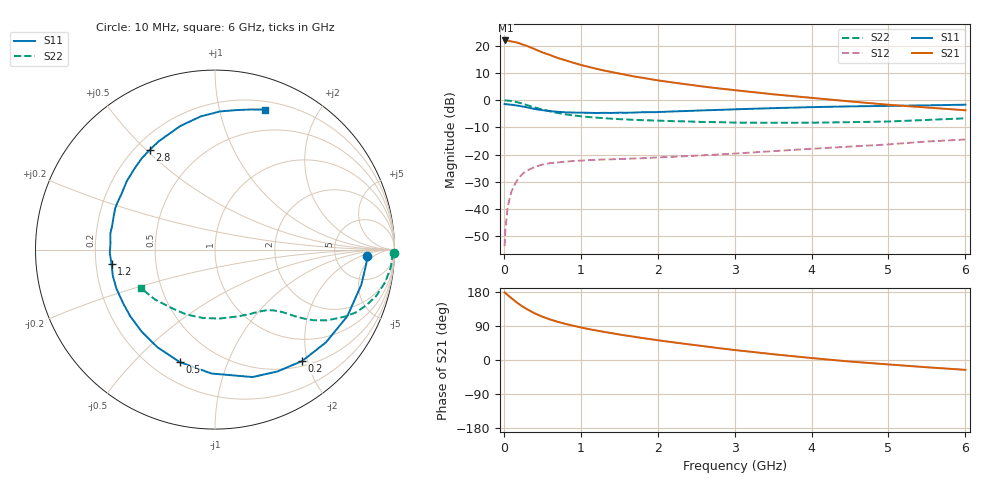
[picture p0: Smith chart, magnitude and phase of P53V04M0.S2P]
! SIEMENS Small Signal Semiconductors
! BFP183
! Si NPN RF Bipolar Junction Transistor in SOT143
! VCE = 3 V  IC = 4 mA
! Common Emitter S-Parameters:  March  1996
# GHz  S  MA  R  50
!  f  S11  S21  S12  S22
! GHz  MAG  ANG  MAG  ANG  MAG  ANG  MAG  ANG
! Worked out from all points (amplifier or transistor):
!   36 points, 10 MHz to 6 GHz, reference 50 ohm
!   highest |S21| = 21.9 dB at 20 MHz (marker M1)
!   |S21| within 3 dB of that: start of sweep to 385.1 MHz
!   unconditionally stable (mu >= 1): 1.679 GHz to 5.723 GHz
!   at 250 MHz: K = 0.18, MSG = 23.6 dB, |S12| = -26.9 dB
!   at 1.4 GHz: K = 0.87, MSG = 16.0 dB, |S12| = -21.7 dB
!   at 6 GHz: K = 0.95, MSG = 5.4 dB, |S12| = -14.4 dB
!   S11 on the Smith chart (normalised r, x): 10 MHz: 12, -3; 200 MHz: 0.58, -1.91; 500 MHz: 0.31, -0.69; 1.2 GHz: 0.27, -0.07; 2.8 GHz: 0.26, +0.51; 6 GHz: 0.28, +1.38
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0.01  0.85 -2.5  12.38 178.5  0.0021 83.7  0.9956 -1.1
0.02  0.8459 -5.6  12.48 177.0  0.0042 86.3  0.989 -2.2
0.05  0.8384 -13.5  12.36 171.2  0.0111 84.3  0.9849 -5.5
0.15  0.8058 -39.9  11.64 154.6  0.0301 69.2  0.935 -16.0
0.2  0.788 -52.0  11.08 147.1  0.0383 63.8  0.8976 -20.3
0.25  0.7629 -62.9  10.42 140.2  0.0454 58.3  0.8585 -24.1
0.3  0.7402 -73.6  9.909 134.3  0.0511 53.7  0.8139 -27.3
0.4  0.6907 -91.6  8.659 123.2  0.0594 46.0  0.7378 -32.3
0.5  0.6568 -107.3  7.544 114.4  0.066 40.4  0.676 -35.6
0.6  0.6316 -120.5  6.746 107.1  0.0701 36.2  0.6247 -37.9
0.7  0.613 -131.8  5.964 100.8  0.0722 33.4  0.582 -39.7
0.8  0.6005 -141.9  5.404 95.3  0.0745 30.7  0.5513 -41.0
1.1  0.5878 -165.5  4.1 81.7  0.0796 26.8  0.4916 -44.2
1.2  0.5818 -171.9  3.782 78.0  0.0805 26.0  0.4794 -45.3
1.5  0.5899 171.5  3.083 67.3  0.0834 25.6  0.4489 -48.6
1.7  0.5939 162.1  2.719 61.2  0.0853 25.6  0.436 -51.4
2.2  0.6223 142.1  2.109 46.7  0.0915 26.6  0.4124 -58.9
2.8  0.6648 123.0  1.642 31.1  0.1012 27.6  0.3952 -70.4
3.5  0.7153 105.7  1.284 15.3  0.1163 28.5  0.385 -86.3
4.5  0.7703 87.9  0.95 -4.1  0.141 26.1  0.3954 -114.0
5.5  0.8052 75.8  0.735 -19.2  0.175 22.3  0.4346 -140.2
6  0.8274 70.5  0.654 -26.0  0.1901 18.4  0.4653 -152.5
